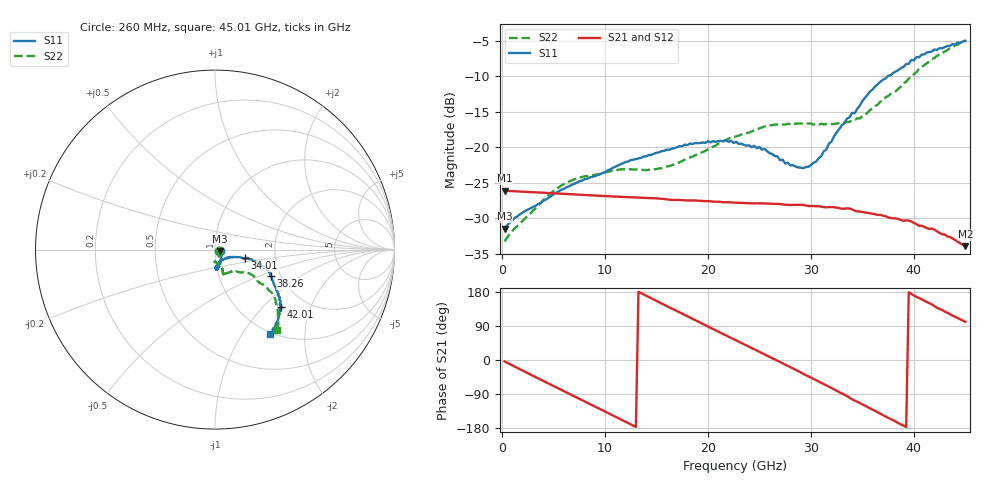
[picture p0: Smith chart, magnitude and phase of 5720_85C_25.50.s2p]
! Device:  ADRF5720
! Description: 0.5dB LSB GaAs MMIC 6-bit Digital Attenuator
! Frequency:  0.000009 -  40 GHz
! Ports:
!	RF1	= Port 1
!	RF2	= Port 2
! Vdd:  3.3 Volt
! Vss:  -3.3 Volt
! Control:  0/3.3 Volt
! State:  25.50 dB attenuation
! Data:  The device was measured using G-S-G Probes on a matrix board.
!  Data was collected using an calibrated 4 port network analyzer.
!  The reference plane for this measurement is at the launchers.
! Note:  Analog Devices supplies this data as a sample of measured data
!  for this product.  Your particular data for this product may vary.
!  Data was taken at 85 degrees C.
!  Analog Devices reserves the right to change this data at anytime.
# GHZ S DB R 45.0
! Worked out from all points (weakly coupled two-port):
!   180 points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, 260 MHz to 45.01 GHz, reference 45 ohm
!   highest |S21| = -26.10 dB at 260 MHz (marker M1); lowest = -33.9 dB at 45.01 GHz (marker M2)
!   lowest |S11| = -31.4 dB at 260 MHz (marker M3), VSWR 1.06, Z = 47.4 - j0.764 ohm
!   |S11| at or under -10 dB: start of sweep to 37.46 GHz
!   |S22| runs from -33.2 to -4.9 dB; largest |S21 - S12| = 0.00027
!   S11 on the Smith chart (normalised r, x): 260 MHz: 1.05, -0.02; 34.01 GHz: 1.40, -0.14; 38.26 GHz: 1.77, -0.59; 42.01 GHz: 1.52, -1.28; 45.01 GHz: 0.97, -1.34
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0.26  -31.44 -17.5  -26.10 -3.8  -26.10 -3.8  -33.25 -22.8
1.26  -29.92 -3.5  -26.19 -17.8  -26.18 -17.7  -31.38 -14.5
5.01  -26.62 -39.1  -26.47 -68.7  -26.45 -68.6  -26.14 -68.2
7.76  -24.71 -53.4  -26.68 -105.7  -26.67 -105.6  -24.18 -83.4
11.51  -22.39 -67.6  -26.97 -156.2  -26.96 -156.2  -23.10 -92.7
15.26  -20.69 -75.6  -27.22 152.4  -27.21 152.6  -22.97 -85.2
18.26  -19.47 -81.3  -27.48 112.2  -27.47 112.4  -21.41 -75.3
22.76  -19.21 -86.6  -27.80 51.5  -27.78 51.7  -18.44 -69.6
25.51  -20.21 -85.5  -27.90 14.8  -27.88 15.1  -17.04 -71.8
28.01  -22.54 -74.1  -28.12 -19.0  -28.11 -18.7  -16.73 -71.5
29.26  -22.93 -54.2  -28.11 -36.3  -28.10 -36.0  -16.60 -71.3
30.26  -22.18 -41.4  -28.26 -49.8  -28.24 -49.5  -16.79 -70.3
31.01  -21.24 -28.6  -28.35 -60.3  -28.33 -60.0  -16.68 -67.8
34.01  -15.14 -16.2  -28.74 -103.7  -28.73 -103.5  -16.19 -52.9
34.26  -15.19 -17.6  -28.93 -107.2  -28.91 -106.9  -16.19 -50.8
36.26  -11.40 -17.8  -29.42 -134.8  -29.40 -134.5  -14.18 -41.0
37.76  -9.82 -22.2  -29.95 -155.9  -29.94 -155.6  -12.46 -34.9
38.26  -9.30 -25.2  -30.00 -162.9  -29.98 -162.5  -12.07 -34.3
40.26  -7.26 -35.0  -30.82 166.5  -30.82 167.0  -9.41 -36.1
42.01  -6.22 -40.9  -31.58 142.1  -31.56 142.1  -7.41 -38.8
43.51  -5.69 -46.9  -32.63 121.1  -32.63 121.4  -6.03 -45.4
45.01  -4.99 -57.0  -33.92 100.6  -33.90 100.9  -4.94 -52.2
